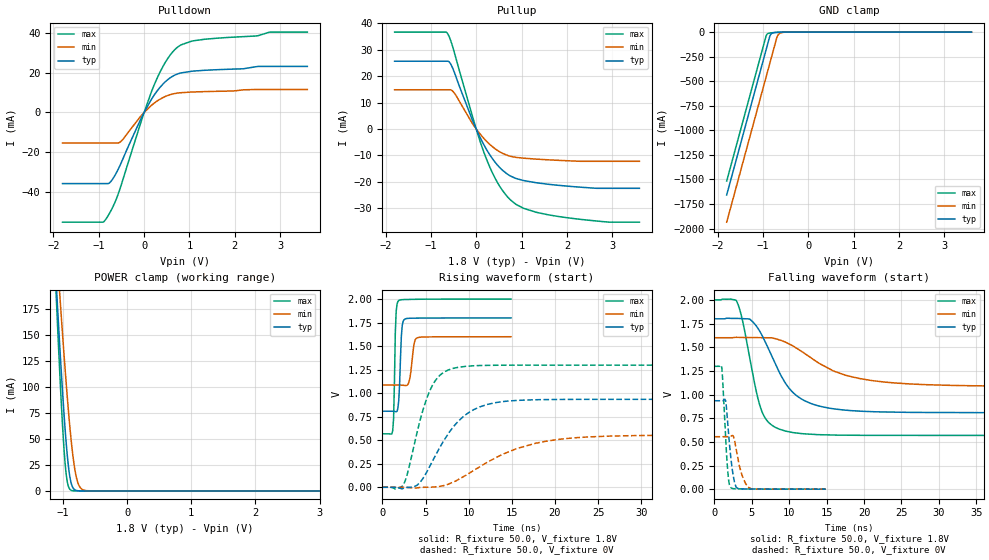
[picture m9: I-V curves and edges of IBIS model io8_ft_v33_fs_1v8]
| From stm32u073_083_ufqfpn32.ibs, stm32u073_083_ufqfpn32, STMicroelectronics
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[Model]   io8_ft_v33_fs_1v8
Model_type I/O
Polarity   Non-Inverting
Enable   Active-Low
| CAP_THRESHOLD on pad IOFT is "UDTCAPC" :
| Rising=30.0% of vddiom   Falling=70.0% of vddiom
| C_comp min and max val. don't necessarily correlate with the min and max pvt
| but are the smallest and greatest pad capacitance found.
| var   typ   min   max
C_comp   2.10717pF  2.10453pF  2.16863pF
|C_comp_pullup   1.19911pF  1.17985pF  1.18490pF
|C_comp_pulldown   908.06325fF  924.67568fF  983.73002fF
Vinl = 480.0mV
Vinh = 1.4V
Vmeas = 900.0mV   | Reference voltage for timing measurements
Cref  = 50.0pF   | Timing specification test load capacitance value
Rref  = 100.0MOhm   | Timing specification test load resistance value
Vref  = 900.0mV   | Timing specification test load voltage
[Model Spec]
| TIME_THRESHOLD on pin ZIV33M is "CMOS" :
| Rising=50.0% of vddiom   Falling=50.0% of vddiom
Vinl 728.70000mV 655.70000mV 817.70000mV
Vinh 1.06430V 949.30000mV 1.16330V
| variable   typ   min   max
[Temperature Range] 25.0 140.0 -40.0
| variable   typ   min   max
[Voltage Range] 1.8V 1.6V 2.0V
| variable   typ   min   max
[POWER Clamp Reference] 1.8V 1.6V 2.0V
| variable   typ   min   max
[GND Clamp Reference] 0V 0V 0V
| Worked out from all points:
|   slope of the pulldown table from 0 to 0.27 V, typ, clamps not added: 26.3 ohm
|   slope of the pullup table from 0 to 0.27 V, typ, clamps not added: 30 ohm
|   GND clamp passes 1 mA (typ) near -0.61 V on its own axis
|   POWER clamp passes 1 mA (typ) near -0.81 V on its own axis
|   rising waveform, R_fixture 50.0, V_fixture 1.8V: 20-80 % time 251ps typ, 394ps min, 200ps max; typ from 0.809 V to 1.8 V
|   falling waveform, R_fixture 50.0, V_fixture 1.8V: 20-80 % time 4.18ns typ, 7.47ns min, 2.26ns max; typ from 1.8 V to 0.809 V
|   rising waveform, R_fixture 50.0, V_fixture 0V: 20-80 % time 4.05ns typ, 7.41ns min, 2.35ns max; typ from 0 V to 0.935 V
|   falling waveform, R_fixture 50.0, V_fixture 0V: 20-80 % time 696ps typ, 1.03ns min, 536ps max; typ from 0.935 V to 0 V
[POWER Clamp]
-1.8V     1.053A     943.1mA    1.262A
-1.11V    202.2mA    242.3mA    190.9mA
-1.09V    180mA      223.6mA    163.4mA
-1.05V    136.9mA    187mA      110.9mA
-980mV    68.91mA    126.1mA    35.23mA
-940mV    37.57mA    94.11mA    10.65mA
-880mV    8.969mA    52.17mA    807.4uA
-830mV    1.697mA    25.82mA    75.79uA
-790mV    394.2uA    12.22mA    11.25uA
-740mV    61.25uA    3.879mA    1.034uA
-660mV    3.073uA    483.4uA    22.7nA
3.6V      0A         0A         0A
[GND Clamp]
-1.8V     -1.658A    -1.935A    -1.517A
-930mV    -179mA     -456mA     -38.91mA
-900mV    -128mA     -405mA     -17.65mA
-850mV    -44.09mA   -320mA     -9.519mA
-830mV    -24.74mA   -286mA     -8.302mA
-790mV    -9.695mA   -218mA     -6.49mA
-700mV    -2.938mA   -65mA      -3.294mA
-670mV    -2.157mA   -31.85mA   -2.435mA
-640mV    -1.545mA   -16.21mA   -1.699mA
-570mV    -571.9uA   -3.807mA   -536.5uA
-420mV    -14.26uA   -143.3uA   -5.434uA
3.6V      449.1pA    102.3nA    316.4pA
| variable   typ   min   max
[Pullup Reference] 1.8V 1.6V 2.0V
| variable   typ   min   max
[Pulldown Reference] 0V 0V 0V
[Pullup]
-1.8V     25.66mA    14.85mA    36.7mA
-630mV    25.66mA    14.85mA    36.09mA
-570mV    24.8mA     14.85mA    33.82mA
-480mV    21.34mA    13.54mA    28.84mA
-90mV     3.62mA     2.224mA    5.223mA
230mV     -7.853mA   -4.702mA   -11.57mA
540mV     -15mA      -8.867mA   -22.31mA
870mV     -18.72mA   -10.75mA   -28.48mA
1.33V     -20.4mA    -11.44mA   -31.6mA
1.9V      -21.5mA    -11.96mA   -33.39mA
2.94V     -22.49mA   -12.26mA   -35.33mA
3.6V      -22.49mA   -12.26mA   -35.33mA
[Pulldown]
-1.8V     -35.76mA   -15.41mA   -55.17mA
-910mV    -35.76mA   -15.41mA   -55.17mA
-830mV    -35.76mA   -15.41mA   -53.18mA
-710mV    -34mA      -15.41mA   -48.42mA
-520mV    -26.05mA   -14.75mA   -37.5mA
-90mV     -4.145mA   -2.306mA   -6.327mA
230mV     8.974mA    4.797mA    14.24mA
490mV     15.87mA    8.223mA    26.01mA
750mV     19.43mA    9.743mA    33.01mA
1.33V     21.16mA    10.45mA    36.75mA
2.78V     23.13mA    11.52mA    40.36mA
3.6V      23.13mA    11.52mA    40.37mA
[Ramp]
dV/dt_r 560.73212mV/4.0464ns 332.41268mV/7.41247ns 778.78246mV/2.34935ns
dV/dt_f 594.84112mV/4.1842ns 308.28523mV/7.47095ns 859.13256mV/2.2558ns
R_load = 50.0
| Removed startup time: 0s 0s 0s  .
| Removed end time: 14.9ns.
[Rising Waveform]
R_fixture   = 50.0
V_fixture   = 1.8V
V_fixture_min = 1.6V
V_fixture_max = 2.0V
0s        808.6mV    1.086V     568.1mV
1.2ns     808.3mV    1.086V     602.2mV
1.3ns     807.6mV    1.086V     728.4mV
1.5ns     804mV      1.086V     1.64V
1.6ns     801.9mV    1.086V     1.869V
1.9ns     923.7mV    1.086V     1.985V
2.2ns     1.606V     1.085V     1.993V
2.6ns     1.786V     1.082V     1.995V
4ns       1.797V     1.586V     1.998V
14.9ns    1.8V       1.6V       2V
| Removed startup time: 0s 0s 0s  .
| Removed end time: 99.9ns.
[Falling Waveform]
R_fixture   = 50.0
V_fixture   = 1.8V
V_fixture_min = 1.6V
V_fixture_max = 2.0V
0s        1.8V       1.6V       2V
2.9ns     1.805V     1.604V     1.995V
3.7ns     1.802V     1.603V     1.8V
4.8ns     1.792V     1.603V     1.352V
6.4ns     1.619V     1.601V     810.2mV
7.8ns     1.381V     1.596V     669mV
10.4ns    1.029V     1.517V     599mV
17.5ns    834.7mV    1.204V     570.1mV
26ns      811.2mV    1.112V     568.1mV
99.9ns    808.6mV    1.086V     568.1mV
| Removed startup time: 0s 0s 0s  .
| Removed end time: 99.9ns.
[Rising Waveform]
R_fixture   = 50.0
V_fixture   = 0V
V_fixture_min = 0V
V_fixture_max = 0V
0s        -9.639uV   -5.556uV   -9.603uV
2.4ns     -12.75mV   178uV      21.19mV
4.1ns     27.89mV    -4.922mV   613.1mV
5.6ns     240.7mV    689.8uV    1.046V
6.8ns     446.2mV    11.68mV    1.201V
8.8ns     701.5mV    81.87mV    1.275V
13.1ns    899mV      312mV      1.297V
17.6ns    929.8mV    464.7mV    1.298V
23.8ns    934.3mV    534.5mV    1.298V
99.9ns    934.6mV    554mV      1.298V
| Removed startup time: 0s 0s 0s  .
| Removed end time: 14.9ns.
[Falling Waveform]
R_fixture   = 50.0
V_fixture   = 0V
V_fixture_min = 0V
V_fixture_max = 0V
0s        934.6mV    554mV      1.298V
1ns       934mV      554mV      1.275V
1.5ns     933.2mV    553.7mV    526.5mV
1.7ns     774.9mV    553.6mV    271.7mV
1.9ns     573.8mV    553.9mV    94mV
2.2ns     324.4mV    559.7mV    15.83mV
2.9ns     21.44mV    420.8mV    3.545mV
3.7ns     2.766mV    144.8mV    2.464mV
4.6ns     1.79mV     16.98mV    1.09mV
14.9ns    80.94uV    253.7uV    19.1uV
